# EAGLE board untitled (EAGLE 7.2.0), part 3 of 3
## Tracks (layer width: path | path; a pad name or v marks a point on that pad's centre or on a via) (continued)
N$276 (continued)
  Bottom 2.184: K10.24 302.16,68.58 K10.14 | K8.1 308.36,68.58 F1.1A F1.1B
N$277
  Bottom 0.406: R115.2 OK8.3
N$278
  Bottom 2.184: F1.2A F1.2B 327.03,65.66 X13.8 334.01,71.12 336.55,73.66 336.55,109.22 334.65,111.12 F2.2A F2.2B
N$279
  Top 0.406: OK8.5 312.42,24.13 323.85,24.13 325.75,26.04 X12.3
N$280
  Top 0.406: OK8.7 317.5,26.67 328.57,26.67 X12.2
N$281
  Top 2.184: R118.2 R117.1
  Bottom 2.184: X13.2 X13.3 | X13.3 X13.4 X13.5 | X13.3 R119.2 313.69,96.52 R117.1
N$282
  Bottom 2.184: K6.1 R117.2 316.23,104.14 318.77,106.68 X13.1
N$283
  Bottom 0.406: IC21.2 229.87,80.01 247.65,80.01 IC22.1
N$284  (via drill 0.6)
  Top 0.406: IC22.2 247.65,78.74 246.38,77.47 v246.38,72.39
  Bottom 0.406: v246.38,72.39 233.68,72.39 232.41,71.12 IC21.5
N$285
  Bottom 0.406: IC21.6 232.41,68.58 233.68,69.85 249.55,69.85 250.19,70.49 250.19,74.93 IC22.3
N$286  (via drill 0.6)
  Top 0.406: IC22.4 248.28,73.66 247.65,73.03 247.65,71.76 246.38,70.49 v246.38,62.87
  Bottom 0.406: v246.38,62.87 245.74,62.23 233.68,62.23 232.41,60.96 IC21.9
N$287  (via drill 0.6)
  Top 0.406: IC22.5 247.65,69.85 247.65,62.23 v246.38,60.96
  Bottom 0.406: v246.38,60.96 IC21.12
N$288
  Bottom 0.406: IC21.15 IC22.6
N$289  (via drill 0.6)
  Top 0.406: v238.76,65.41 v238.76,71.12
  Bottom 0.406: IC22.7 248.28,65.41 243.2,65.41 242.57,64.77 239.39,64.77 v238.76,65.41 | v238.76,71.12 IC21.16
N$290
  Bottom 0.406: IC21.19 241.3,78.74 242.57,77.47 250.19,77.47 251.46,76.2 251.46,68.58 250.19,67.31 250.19,64.77 IC22.8
N$291
  Bottom 0.406: SV3.1 114.62,64.45 109.22,69.85 95.89,69.85 95.25,69.22 95.25,68.26 94.3,67.31 93.34,67.31 89.85,63.82 86.36,63.82 85.09,62.55 85.09,46.99 IC23.35
N$292  (via drill 0.6)
  Top 0.406: IC15.15 148.59,26.67 v147.32,27.94 | v100.65,28.89 97.79,31.75 97.79,40.32 92.71,45.4 92.71,48.58 91.76,49.53 91.12,49.53 91.12,68.26 IC23.64
  Bottom 0.406: v147.32,27.94 147,28.26 101.28,28.26 v100.65,28.89
N$293
  Top 0.406: IC24.2 85.41,12.7 89.22,12.7 90.49,13.97 90.49,42.86 88.9,44.45 IC23.39
N$294
  Top 0.61: R120.2 IC24.4
N$295
  Bottom 0.406: IC24.1 86.68,15.24 86.04,15.88 84.77,15.88 84.14,16.51 R121.2
N$296
  Top 0.406: SV4.2 IC24.7
N$297  (via drill 0.6)
  Top 0.406: IC24.3 80.33,15.24 v80.33,37.47 | v74.3,38.1 75.25,39.05 75.25,44.77 IC23.29
  Bottom 0.406: v80.33,37.47 79.69,38.1 v74.3,38.1
N$298
  Top 0.406: IC24.8 SV4.4
N$299
  Bottom 0.406: IC24.5 80.33,5.08 82.87,5.08 SV4.3
  Bottom 0.61: C61.1 SV5.3 89.85,1.91 86.04,1.91 SV4.3
N$300
  Top 0.406: SV4.1 IC24.6
N$301
  Bottom 0.61: SV5.4 C61.2
N$302
  Top 0.406: IC25.2 76.52,37.47 79.06,40.01 80.33,40.01 80.33,44.13 IC23.31
  Bottom 0.406: SV6.9 62.86,44.45 63.82,43.5 78.11,43.5 78.74,44.13 IC23.31
N$303
  Bottom 0.406: IC25.4 IC25.3 79.06,35.56 78.42,36.2 73.66,36.2 71.75,38.1 R122.1
N$304  (via drill 0.6)
  Top 0.406: SV6.8 68.58,50.8 69.85,49.53 74.93,49.53 IC23.30 | R122.2 v69.85,45.4
  Bottom 0.406: v69.85,45.4 66.67,45.4 66.67,49.53 SV6.8
N$305
  Top 0.406: IC25.1 73.98,36.2 77.79,40.01 77.79,44.13 77.47,44.45 77.47,46.99 IC23.32
  Bottom 0.406: SV6.10 65.41,44.77 65.72,44.45 76.84,44.45 77.47,45.09 77.47,46.99 IC23.32
N$306
  Top 0.406: IC26.8 IC26.1
N$307
  Top 0.406: IC26.7 60.33,41.28 U$2.C
N$308
  Top 0.406: IC26.6 63.5,42.86 64.14,43.5 66.99,43.5 68.9,45.4 68.9,46.04 69.85,46.99 71.75,46.99 73.03,48.26 IC23.28
N$309
  Top 0.61: X14.4 53.14,7.42 55.88,10.16 IC27.13
N$310
  Top 0.61: X14.3 55.88,7.62 58.42,10.16 IC27.14
N$311  (via drill 0.6)
  Top 0.406: IC27.12 53.34,15.24 50.8,17.78 49.53,17.78 46.99,20.32 v46.99,25.4 | v46.99,30.48 48.26,31.75 48.26,36.83 57.15,45.72 v57.15,61.6 | IC23.17 72.39,59.69 68.58,59.69 v66.67,61.6
  Bottom 0.406: v46.99,25.4 v46.99,30.48 | v57.15,61.6 v66.67,61.6
N$312  (via drill 0.6)
  Top 0.406: IC27.11 48.26,16.51 46.99,16.51 43.18,20.32 v43.18,25.4 | v43.18,30.48 43.18,29.21 44.45,27.94 48.26,27.94 49.53,29.21 49.53,36.83 58.42,45.72 v58.42,60.33 | IC23.18 68.58,58.42 v66.67,60.33
  Bottom 0.406: v43.18,25.4 v43.18,30.48 | v58.42,60.33 v66.67,60.33
N$313
  Bottom 0.406: IC27.3 58.42,22.86 59.69,24.13 63.82,24.13 C62.-
N$314
  Bottom 0.406: IC27.1 67.31,25.4 67.63,25.4 C62.+
N$315
  Top 0.406: IC27.4 55.88,25.08 C63.+
N$316
  Top 0.406: IC27.5 53.34,25.08 C63.-
N$317
  Top 0.406: IC27.6 C64.-
N$318  (via drill 0.6)
  Top 0.406: v125.73,12.7 125.73,20 v125.41,20.32 | v95.25,17.78 v95.25,27.94 | v74.93,27.94 74.93,29.53 72.39,32.07 72.39,42.86 74.93,45.4 74.93,46.36 75.25,46.67 76.2,46.67 77.47,47.94 v77.47,49.53 | v77.47,52.07 77.47,62.23 76.2,63.5 IC23.15
  Bottom 0.406: IC15.42 160.34,11.43 159.07,10.16 149.86,10.16 147.32,12.7 v125.73,12.7 | v125.41,20.32 118.11,20.32 115.57,17.78 v95.25,17.78 | v95.25,27.94 v74.93,27.94 | v77.47,49.53 v77.47,52.07
N$319
  Top 0.406: C65.+ IC27.2
N$320
  Top 0.406: IC23.19 72.39,57.15 64.14,57.15 SV6.3
N$321
  Top 0.406: SV6.4 IC23.20
N$322
  Top 0.406: IC23.21 72.39,54.61 64.14,54.61 SV6.5
N$323
  Top 0.406: IC23.22 SV6.6
N$324
  Top 0.406: IC23.23 72.39,52.07 64.14,52.07 SV6.7
N$325
  Bottom 0.406: IC23.67 86.36,72.39 81.6,77.15 QF1.3 82.55,79.82 C70.2
N$326
  Bottom 0.406: IC23.66 87.63,69.85 85.73,69.85 85.09,70.49 85.09,72.39 81.28,76.2 76.01,76.2 QF1.1 72.39,79.82 C69.2
N$327
  Top 1.676: X15.1 7.62,104.14 7.62,124.46 | 7.62,124.46 10.16,124.46 | 7.62,124.46 F3.1A
N$328
  Bottom 1.676: B2.AC2 F4.2A 30.48,83.82
N$329
  Bottom 2.184: X15.9 13.97,63.5 15.87,61.6 15.87,48.64 F5.1A
N$330
  Top 0.406: C79.1 20.32,114.3 C78.+
  Top 1.676: C78.+ 19.05,107.95 19.05,104.14 17.78,102.87 17.78,96.52 19.05,95.25 IC28.IN
  Bottom 1.676: B1.+ 10.16,116.84 15.24,116.84 | 15.24,116.84 17.78,116.84 C78.+ | D50.C 15.24,116.84 | IC28.IN 24.13,92.71 27.94,92.71 29.21,91.44 D46.C
N$331
  Top 0.406: D47.A 33.02,103.12
  Top 1.676: C80.- 33.02,103.12 32.77,103.12 30.48,105.41 C78.- | X15.4 12.7,88.9 12.7,104.14 D50.A
  Bottom 0.406: C79.2 22.86,119.38 C78.- | 5.08,88.9 C81.2
  Bottom 1.676: C80.- 34.29,101.6 30.48,97.79 IC28.GND 19.05,97.79 12.7,91.44 12.7,88.9 X15.4 5.08,88.9
  Bottom 1.778: B1.- 7.62,113.03 12.7,113.03 15.24,110.49 D50.A
N$332
  Top 0.406: D47.K 33.02,91.44 34.29,90.17 R123.2
N$333
  Top 0.406: C80.+ 35.81,103.89 36.83,102.87 R123.1
  Bottom 0.406: 5.08,93.98 C81.1
  Bottom 1.676: C80.+ 31.75,105.09 D46.A 24.13,102.87 IC28.OUT 17.78,100.33 11.43,93.98 X15.3 5.08,93.98
N$334
  Bottom 1.676: X15.5 F4.1A 20.32,83.82
N$335
  Top 0.406: C83.1 21.59,71.12 D51.C
  Top 1.676: B2.+ 45.72,83.82 44.45,82.55 44.45,73.66 39.37,68.58 C82.+
  Bottom 1.676: C82.+ 25.4,68.58 D51.C 19.05,62.23 19.05,54.61 20.32,53.34 IC29.IN 24.13,50.8 D48.C
N$336
  Bottom 2.184: F5.2A 34.29,45.72 30.48,41.91 6.91,41.91 B3.AC1
N$337
  Bottom 2.184: X15.10 11.43,58.42 12.06,57.79 12.06,50.17 9.08,47.18 B3.AC2
N$338  (via drill 0.6)
  Top 0.813: v43.18,64.77 43.18,43.18 40.01,40.01 27.3,40.01 R127.1 | D53.C 21.59,19.05
  Top 1.27: 21.59,27.94 21.59,19.05 IC30.3
  Top 2.184: D52.C 21.59,27.94 26.67,27.94 C86.+
  Bottom 0.813: R24.1 55.88,93.98 55.25,94.62 49.53,94.62 48.9,93.98 48.9,76.84 43.18,71.12 v43.18,64.77
  Bottom 1.422: C87.1 22.86,39.37 R127.1 30.48,35.56 SV7.1
  Bottom 1.93: C86.+ 30.48,35.56
  Bottom 2.184: D52.C 10.16,27.94 6.67,31.43 B3.+
N$339
  Bottom 0.406: R127.2 D54.K
N$340
  Bottom 0.406: D49.K R124.2
N$341
  Bottom 2.184: 19.05,45.72 24.13,45.72
N$342
  Bottom 0.406: R125.2 R126.1 IC30.1

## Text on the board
Top: Isel IMC4 Layout | < +28V | GND | EE2506_1 | 1.25A T | BS | PLT-Nr . #568120 V1 .6 | 1.25A TRAEGE | 1.25A T | ISEL AUTOMATION | 5A TRAEGE | 1.25A T | BS | Gabs'e 2015 | !!! ACHTUNG Es wird keine Haftung für die / Richtigkeit von Schaltplan und Layout übernommen !!!
Bottom: LS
